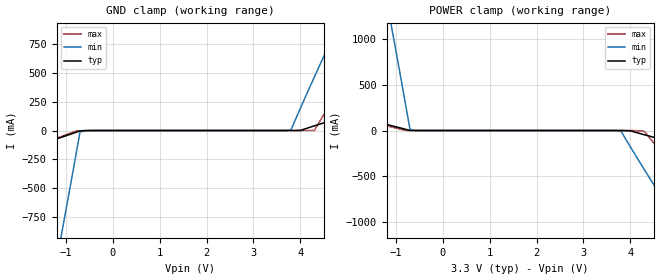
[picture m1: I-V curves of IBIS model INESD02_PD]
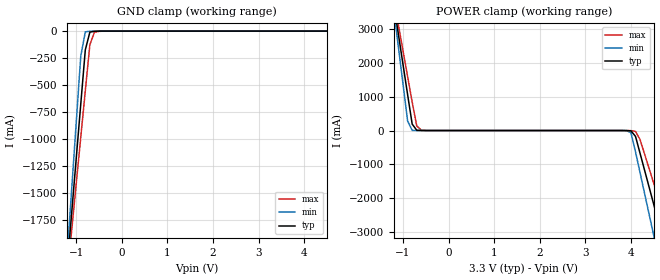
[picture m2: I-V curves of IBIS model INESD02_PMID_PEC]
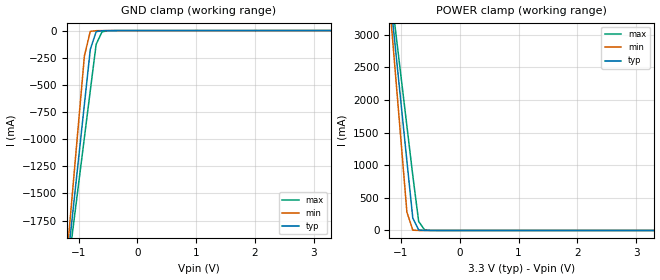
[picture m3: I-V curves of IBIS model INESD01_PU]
|   This file is an IBIS representation of the   |
|   Integrated Device Technology, Inc.   |
|   ICS831742I   |
|   DIFFERENTIAL CLOCK/DATA MULTIPLEXER   |
[IBIS Ver]   4.1
[File name]   831742i_3v3.ibs
[File Rev]   1.1
|1.1
|Added zero crossing point to output Pullup IV data.
|29 Jun 2012
|1.0
|Original Model
[Date]   21 Feb 2016
[Source]   Originated at Integrated Device Technology, Inc.
[Disclaimer]
IDT hereby grants the user of this IBIS model a non-exclusive,
nontransferable license to use this IBIS model under the following terms.
Before using this IBIS model, the user should read this license.
If the user does not accept these terms,  the IBIS model should be
returned to IDT within 30 days.
   The user is granted this license only to use the IBIS model and
is not granted rights to sell, load, rent, lease or license the IBIS
model in whole or in part, or in modified form to anyone other than
user. User may modify the IBIS model to suit its specific
applications but rights to derivative works and such modifications
shall belong to IDT.
   This IBIS model is provided on an "AS IS" basis and IDT makes
absolutely no warranty with respect to the information contained
herein. IDT DISCLAIMS AND CUSTOMER WAIVES ALL WARRANTIES, EXPRESS
OR IMPLIED, INCLUDING WARRANTIES OF MERCHANTABILITY OR FITNESS FOR
A PARTICULAR PURPOSE. The entire risk as to quality and performance
is with the Customer. ACCORDINGLY, IN NO EVENT SHALL THE COMPANY BE
LIABLE FOR ANY DAMAGES, WHETHER IN CONTRACT OR TORT,INCLUDING ANY
LOST PROFITS OR OTHER INCIDENTAL, CONSEQUENTIAL, EXEMPLARY, OR
PUNITIVE DAMAGES ARISING OUT OF THE USE OR APPLICATION OF THE IBIS
model provided in this package. Further, IDT reserves the right to
make changes without notice to any product herein to improve
reliability, function, or design. IDT does not convey any license
under patent rights or any other intellectual property rights,
including those of third parties.
   IDT is not obligated to provide maintenance or support
for the licensed IBIS model.
[Copyright] Copyright 2012 by Integrated Device Technology, Inc.
[Component]   ICS831742GI
[Manufacturer] Integrated Device Technology, Inc.
[Package]
|TSSOP 24 Lead
|   typ   min   max
R_pkg   60.65m   52.4m   68.9m
L_pkg   1.989nH   1.431nH   2.547nH
C_pkg   0.314pF   0.254pF   0.374pF
[Pin] signal_name   model_name   R_pin   L_pin   C_pin
1   GND   GND   68.9m   2.547n   0.374p
2   CLK0   INESD02_PD   65.6m   2.323n   0.350p
3   nCLK0   INESD02_PMID_PEC   62.3m   2.100n   0.326p
4   VDD   POWER   59.0m   1.877n   0.302p
5   CLK1   INESD02_PD   55.7m   1.654n   0.278p
6   nCLK1   INESD02_PMID_PEC   52.4m   1.431n   0.254p
7   CLK2   INESD02_PD   52.4m   1.431n   0.254p
8   nCLK2   INESD02_PMID_PEC   55.7m   1.654n   0.278p
9   GND   GND   59.0m   1.877n   0.302p
10   CLK3   INESD02_PD   62.3m   2.100n   0.326p
11   nCLK3   INESD02_PMID_PEC   65.6m   2.323n   0.350p
12   VDD   POWER   68.9m   2.547n   0.374p
13   nOEA   INESD01_PU   68.9m   2.547n   0.374p
14   nOEB   INESD01_PU   65.6m   2.323n   0.350p
15   VDD   POWER   62.3m   2.100n   0.326p
16   SEL   INESD01_PD   59.0m   1.877n   0.302p
17   QA   DCMOUT01_ISO2_PM   55.7m   1.654n   0.278p
18   nQA   DCMOUT01_ISO2_PM   52.4m   1.431n   0.254p
19   QB   DCMOUT01_ISO2_PM   52.4m   1.431n   0.254p
20   nQB   DCMOUT01_ISO2_PM   55.7m   1.654n   0.278p
21   VDD   POWER   59.0m   1.877n   0.302p
22   SEL0   INESD01_PD   62.3m   2.100n   0.326p
23   IREF   NC   65.6m   2.323n   0.350p
24   SEL1   INESD01_PD   68.9m   2.547n   0.374p
[Diff Pin]  inv_pin  vdiff tdelay_typ tdelay_min  tdelay_max
2   3   0.15   NA   NA   NA
5   6   0.15   NA   NA   NA
10   11   0.15   NA   NA   NA
17   18   NA   0   0   0
19   20   NA   0   0   0
| Models and submodels in the file (5): INESD02_PD (Input), INESD02_PMID_PEC (Input), INESD01_PU (Input), INESD01_PD (Input), DCMOUT01_ISO2_PM (Open_source)
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[Model]   INESD02_PD
Model_type   Input
Polarity   Non-Inverting
Vinl = 0.8V
Vinh = 2.0V
|   typ   min   max
C_comp   2pF   1.5pF   2.5pF
|   typ   min   max
[Voltage range]   3.3V   3.135V   3.465V
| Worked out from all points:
|   GND clamp passes 1 mA (typ) near -0.60 V on its own axis
|   POWER clamp passes 1 mA (typ) near -0.70 V on its own axis
[GND_clamp]
|Voltage   I (typ)   I (min)   I (max)
-3.3V     -332.3mA   -5.292A    -346.3mA
-2.2V     -203.6mA   -3.226A    -207.3mA
-1.1V     -59.83mA   -918.6mA   -51.9mA
-1V       -45.96mA   -695.9mA   -36.91mA
-700mV    -3.491mA   -14.25mA   -2.553mA
-500mV    -180.1uA   -382.8uA   -57.92uA
3.8V      83.75uA    4.893mA    57.37uA
4V        862uA      192.6mA    61.17uA
4.3V      40.69mA    467.1mA    1.452mA
4.8V      104.5mA    906.7mA    336.6mA
5.7V      211.5mA    1.644A     899.1mA
6.6V      309.2mA    2.318A     1.413A
[Power_clamp]
|Voltage   I (typ)   I (min)   I (max)
-3.3V     309.2mA    6.635A     293.4mA
-1.1V     53.7mA     1.148A     39.81mA
-1V       40.69mA    868.5mA    26.9mA
-800mV    14.27mA    301.3mA    677.5uA
-700mV    862uA      13.32mA    132.7uA
-500mV    83.75uA    187.9uA    60.1uA
3.8V      -180.1uA   -6.224mA   -5.27uA
4V        -3.491mA   -176.5mA   -129.9uA
4.3V      -45.96mA   -425.6mA   -8.439mA
5.2V      -165.9mA   -1.129A    -564.9mA
6.2V      -287.1mA   -1.84A     -1.127A
6.6V      -332.3mA   -2.105A    -1.336A
[Model]   INESD02_PMID_PEC
Model_type   Input
Polarity   Non-Inverting
Vinl = 0.8V
Vinh = 2.0V
|   typ   min   max
C_comp   2pF   1.5pF   2.5pF
|   typ   min   max
[Voltage range]  3.3V   3.135V   3.465V
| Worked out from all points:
|   GND clamp passes 1 mA (typ) near -0.54 V on its own axis
|   POWER clamp passes 1 mA (typ) near -0.60 V on its own axis
[GND_clamp]
|Voltage   I(typ)   I(min)   I(max)
-3.3V     -12.83A    -15.14A    -11.37A
-1.2V     -2.195A    -2.092A    -2.281A
-1.1V     -1.689A    -1.472A    -1.849A
-900mV    -678.6mA   -232.7mA   -984.9mA
-800mV    -174mA     -7.255mA   -553.3mA
-700mV    -9.789mA   -1.13mA    -126.1mA
-600mV    -1.72mA    -254.4uA   -11.17mA
-500mV    -427uA     -99.72uA   -2.216mA
6.6V      76.52uA    70.16uA    79.2uA
[POWER_clamp]
|Voltage   I(typ)   I(min)   I(max)
-3.3V     22.38A     26.45A     19.82A
-1.2V     3.723A     3.545A     3.874A
-1.1V     2.836A     2.457A     3.116A
-900mV    1.063A     281mA      1.601A
-800mV    191.6mA    5.071mA    844mA
-600mV    678.1uA    76.63uA    10.7mA
3.9V      -1.629mA   -3.157mA   -831.1uA
4.1V      -173.9mA   -635.2mA   -23.94mA
4.5V      -2.195A    -3.116A    -1.568A
4.7V      -3.206A    -4.358A    -2.433A
4.9V      -4.218A    -5.6A      -3.298A
6.6V      -12.83A    -16.16A    -10.66A
[Model]   INESD01_PU
Model_type   Input
Polarity   Non-Inverting
Vinl = 0.8V
Vinh = 2.0V
|   typ   min   max
C_comp   2pF   1.5pF   2.5pF
|   typ   min   max
[Voltage range]  3.3V   3.135V   3.465V
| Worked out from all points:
|   GND clamp passes 1 mA (typ) near -0.55 V on its own axis
|   POWER clamp passes 1 mA (typ) near -0.61 V on its own axis
[GND_clamp]
|Voltage   I(typ)   I(min)   I(max)
-3.3V     -12.83A    -15.14A    -11.37A
-1.2V     -2.195A    -2.092A    -2.281A
-1.1V     -1.689A    -1.472A    -1.849A
-900mV    -678.5mA   -232.7mA   -984.8mA
-800mV    -174mA     -7.237mA   -553.3mA
-700mV    -9.767mA   -1.114mA   -126.1mA
-600mV    -1.7mA     -240.1uA   -11.15mA
-300mV    -81.66uA   -67.79uA   -163.4uA
3.3V      1.866nA    1.113pA    239.1nA
[POWER_clamp]
|Voltage   I(typ)   I(min)   I(max)
-3.3V     22.38A     26.45A     19.82A
-1.2V     3.723A     3.545A     3.874A
-1.1V     2.836A     2.457A     3.116A
-1V       1.949A     1.369A     2.358A
-900mV    1.063A     281mA      1.601A
-800mV    191.5mA    5.012mA    843.9mA
-700mV    8.032mA    142.2uA    138.3mA
-600mV    607uA      17.63uA    10.62mA
-400mV    16.32uA    7.545uA    335.9uA
3.3V      -71.13uA   -62.11uA   -78.26uA
